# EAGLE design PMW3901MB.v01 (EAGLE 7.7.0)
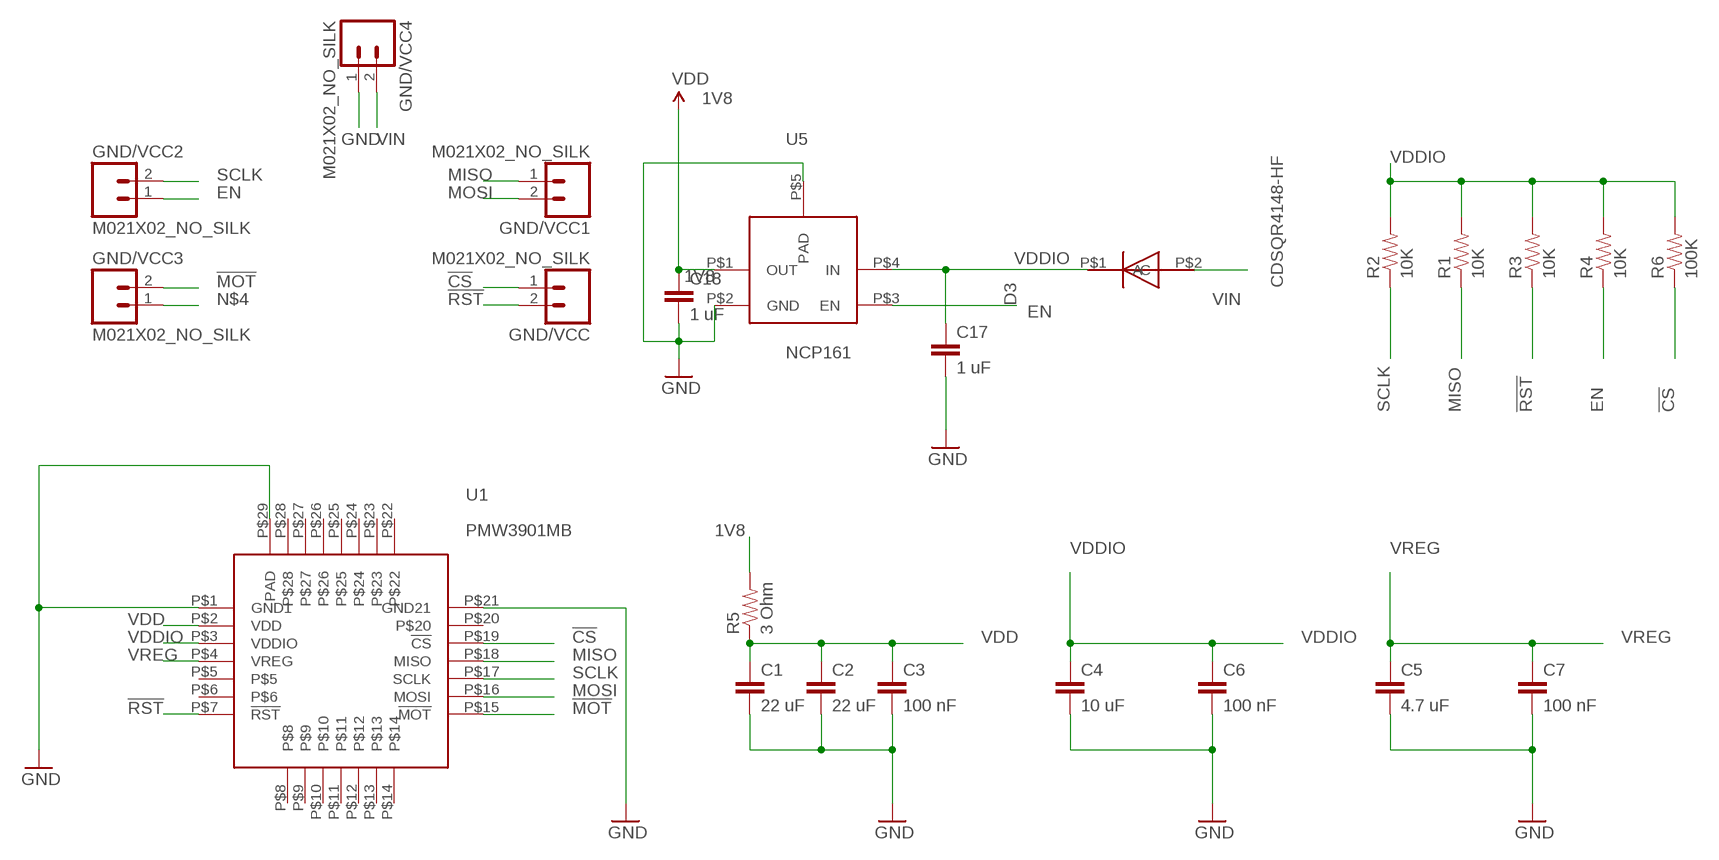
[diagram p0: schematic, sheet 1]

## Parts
C1  22 uF  0402CAP.KW  [0402-CAP@1]
C2  22 uF  0402CAP.KW  [0402-CAP@1]
C3  100 nF  0402CAP.KW  [0402-CAP@1]
C4  10 uF  0402CAP.KW  [0402-CAP@1]
C5  4.7 uF  0402CAP.KW  [0402-CAP@1]
C6  100 nF  0402CAP.KW  [0402-CAP@1]
C7  100 nF  0402CAP.KW  [0402-CAP@1]
C17  1 uF  0402CAP.KW  [0402-CAP@1]
C18  1 uF  0402CAP.KW  [0402-CAP@1]
D3  CDSQR4148-HF  [CDSQR4148-HF]
GND/VCC  M021X02_NO_SILK  [1X02_NO_SILK]
GND/VCC1  M021X02_NO_SILK  [1X02_NO_SILK]
GND/VCC2  M021X02_NO_SILK  [1X02_NO_SILK]
GND/VCC3  M021X02_NO_SILK  [1X02_NO_SILK]
GND/VCC4  M021X02_NO_SILK  [1X02_NO_SILK]
R1  10K  0402RES.KW  [0402-RES]
R2  10K  0402RES.KW  [0402-RES]
R3  10K  0402RES.KW  [0402-RES]
R4  10K  0402RES.KW  [0402-RES]
R5  3 Ohm  0402RES.KW  [0402-RES]
R6  100K  0402RES.KW  [0402-RES]
U1  PMW3901MB  [PMW3901MB]
U5  NCP161  [NCP161]

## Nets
1V8: C18.1 R5.2 U5.P$1(OUT) ; supply symbol labelled VDD
!CS: GND/VCC.1 R6.1 U1.P$19(!CS)
!MOT: GND/VCC3.2 U1.P$15(!MOT)
!RST: GND/VCC.2 R3.1 U1.P$7(!RST)
EN: GND/VCC2.1 R4.1 U5.P$3(EN)
GND: C1.2 C2.2 C3.2 C4.2 C5.2 C6.2 C7.2 C17.2 C18.2 GND/VCC4.1 U1.P$1(GND1) U1.P$21(GND21) U1.P$29(PAD) U5.P$2(GND) U5.P$5(PAD)
MISO: GND/VCC1.1 R1.1 U1.P$18(MISO)
MOSI: GND/VCC1.2 U1.P$16(MOSI)
N$4: GND/VCC3.1
SCLK: GND/VCC2.2 R2.1 U1.P$17(SCLK)
VDD: C1.1 C2.1 C3.1 R5.1 U1.P$2(VDD)
VDDIO: C4.1 C6.1 C17.1 D3.P$1(C) R1.2 R2.2 R3.2 R4.2 R6.2 U1.P$3(VDDIO) U5.P$4(IN)
VIN: D3.P$2(A) GND/VCC4.2
VREG: C5.1 C7.1 U1.P$4(VREG)
Unconnected: U1.P$5 U1.P$6 U1.P$8 U1.P$9 U1.P$10 U1.P$11 U1.P$12 U1.P$13 U1.P$14 U1.P$20 U1.P$22 U1.P$23 U1.P$24 U1.P$25 U1.P$26 U1.P$27 U1.P$28

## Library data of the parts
C1-C7 C17 C18 = SparkFun-Capacitors:0402CAP.KW
D3 = kris:CDSQR4148-HF: ComChip's CDSQR4148-HF high speed 150 mA Io diode
GND/VCC GND/VCC1-GND/VCC4 = SparkFun-Connectors:M02: Standard 2-pin 0.1" header. Use with
R1-R6 = SparkFun-Resistors:0402RES.KW
U1 = kris:PMW3901MB: PMW3901MB flow control camera https://wiki.bitcraze.io/_media/projects:crazyflie2:expansionboards:pot0189-pmw3901mb-txqt-ds-r1.00-200317_20170331160807_public.pdf
U5 = kris:NCP161: NCP161 3V3 LDO voltage regulator

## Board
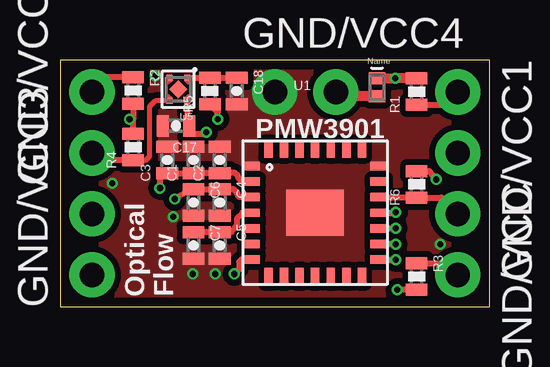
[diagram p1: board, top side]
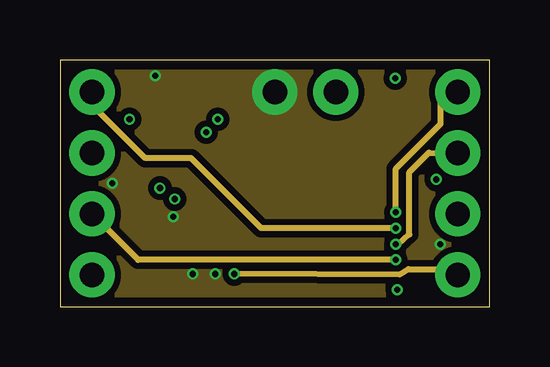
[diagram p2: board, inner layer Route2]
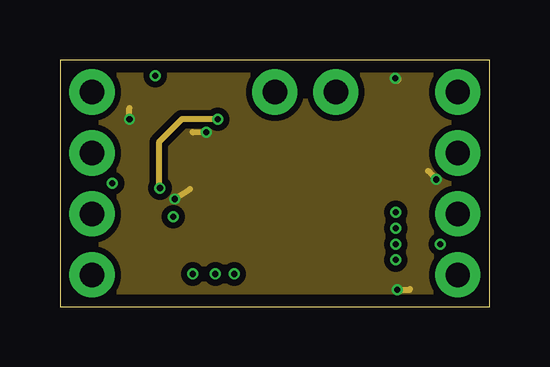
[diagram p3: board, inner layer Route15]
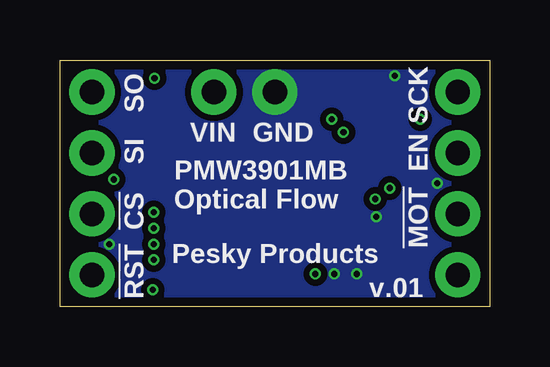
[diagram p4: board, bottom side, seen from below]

Size 17.91 x 10.29 mm. Coordinates in mm from the lower left corner, seen from the top.
Outline: 0,0 17.91,0 17.91,10.29 0,10.29 0,0
Copper layers (1*2*15*16): Top 0.035559375mm / dielectric 0.17018125mm / Route2 0.01778125mm / dielectric 47mil / Route15 0.01778125mm / dielectric 0.17018125mm / Bottom 0.035559375mm
Design rules "OSHPark-4layer *": minimum track width 5mil, minimum drill 10mil, track to track 5mil, track to pad 5mil, pad to pad 5mil, via to via 5mil, smd to smd 5mil, copper to edge 15mil, drill to drill 6mil, minimum pad ring 4mil, minimum via ring 4mil, stop-mask expansion 2.5mil, vias tented up to drill 20mil, thermal gap 10mil

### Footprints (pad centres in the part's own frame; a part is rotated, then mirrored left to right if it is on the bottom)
0402-CAP@1 = smd 0.5 x 0.9: 1 -0.55,0; 2 0.55,0
CDSQR4148-HF = smd 0.7 x 0.5: P$1 0,0.375; P$2 0,-0.375
1X02_NO_SILK = drill 1.016 pad 1.88: 1 0,0; 2 2.54,0
0402-RES = smd 0.5 x 0.9: 1 -0.55,0; 2 0.55,0
PMW3901MB = smd 0.7 x 0.35: P$1 -2.65,1.95; P$2 -2.65,1.3; P$3 -2.65,0.65; P$4 -2.65,0; P$5 -2.65,-0.65; P$6 -2.65,-1.3; P$7 -2.65,-1.95; P$15 2.65,-1.95; P$16 2.65,-1.3; P$17 2.65,-0.65; P$18 2.65,0; P$19 2.65,0.65; P$20 2.65,1.3; P$21 2.65,1.95 | smd 0.35 x 0.7: P$8 -1.95,-2.65; P$9 -1.3,-2.65; P$10 -0.65,-2.65; P$11 0,-2.65; P$12 0.65,-2.65; P$13 1.3,-2.65; P$14 1.95,-2.65; P$22 1.95,2.65; P$23 1.3,2.65; P$24 0.65,2.65; P$25 0,2.65; P$26 -0.65,2.65; P$27 -1.3,2.65; P$28 -1.95,2.65 | smd 2.4 x 1.9: P$29 0,0
NCP161 = smd 0.24 x 0.24: P$1 -0.37,-0.48; P$2 0.37,-0.48; P$3 0.37,0.48; P$4 -0.37,0.48 | smd 0.52 x 0.52 rotated 45: P$5 0,0

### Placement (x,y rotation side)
C1  5.56,6.12 90 top
C2  6.65,6.12 90 top
C3  4.47,6.12 90 top
C4  6.65,4.34 270 top
C5  6.65,2.57 270 top
C6  5.56,4.34 270 top
C7  5.56,2.57 270 top
C17  4.83,7.54 180 top
C18  7.37,8.99 270 top
D3  13.21,9.14 0 top
GND/VCC  16.57,3.87 270 top
GND/VCC1  16.57,8.95 270 top
GND/VCC2  1.33,6.41 90 top
GND/VCC3  1.33,1.33 90 top
GND/VCC4  8.95,8.95 0 top
R1  14.86,8.97 90 top
R2  3.05,9.02 270 top
R3  14.86,1.27 270 top
R4  3.05,6.65 90 top
R5  6.25,8.99 90 top
R6  14.86,5.11 90 top
U1  10.63,3.92 0 top
U5  4.93,9.07 180 top

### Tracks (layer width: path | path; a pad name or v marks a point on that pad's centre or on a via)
1V8
  Top 0.254: U5.P$1 R5.2 C18.1
!CS
  Top 0.254: U1.P$19 14.84,4.57 R6.1 15.89,4.55 GND/VCC.1
!MOT  (via drill 0.25)
  Top 0.254: U1.P$15 13.98,1.97 v13.99,1.96
  Route2 0.254: v13.99,1.96 3.25,1.96 GND/VCC3.2
!RST  (via drill 0.25)
  Top 0.254: R3.1 16.09,1.82 GND/VCC.2 | U1.P$7 7.56,1.97 7.47,1.88 7.47,1.57 v7.26,1.37
  Route2 0.254: v7.26,1.37 14.15,1.35 14.53,1.57 16.33,1.57 GND/VCC.2
EN
  Top 0.203: U5.P$3 3.96,8.59 3.73,8.36 3.73,6.27 3.56,6.11 R4.1
  Top 0.254: R4.1 1.64,6.11 GND/VCC2.1
  Route2 0.254: 1.35,6.43 GND/VCC2.1
GND  (via drill 0.25)
  other vias: 3.96,9.63 15.85,2.62 5.54,1.37 6.48,1.37 4.72,3.76 2.18,5.16
  pour Bottom (isolate 0.254, no thermals): 0,10.29 17.78,10.16 17.78,0 0,0
  pour Top (isolate 0.254, no thermals): 0,10.29 17.78,10.16 17.78,0 0,0
  pour Route2 (isolate 0.254, no thermals): 0,10.29 17.78,10.16 17.78,0 0,0
MISO  (via drill 0.25)
  Top 0.254: R1.1 16.04,8.42 GND/VCC1.1 | U1.P$18 14.11,3.92 v13.99,3.94
  Route2 0.254: v13.99,3.94 13.99,5.77 15.85,7.62 15.85,8.94 16.2,8.59 GND/VCC1.1
MOSI  (via drill 0.25)
  Top 0.254: U1.P$16 13.78,2.62 v13.99,2.62
  Route2 0.254: v13.99,2.62 14.1,2.62 14.55,3.02 14.55,5.61 15.37,6.43 GND/VCC1.2
SCLK  (via drill 0.25)
  Top 0.254: R2.1 1.95,9.57 GND/VCC2.2 | U1.P$17 13.94,3.27 v13.99,3.28
  Route2 0.254: v13.99,3.28 8.38,3.28 5.46,6.2 3.56,6.2 1.4,8.33 1.4,8.89 GND/VCC2.2
VDD  (via drill 0.25)
  Top 0.254: U1.P$2 7.58,5.22 7.42,5.38 7.42,5.46 7.29,5.59 6.7,5.59 C2.1 C1.1 C3.1 4.17,5.41 v4.17,4.95 | v6.58,7.82 6.58,8.11 R5.1
  Route15 0.254: v6.58,7.82 5.08,7.82 4.12,6.86 4.12,5 v4.17,4.95
VDDIO  (via drill 0.25)
  Top 0.203: 5.3,7.65 C17.1
  Top 0.254: U1.P$3 7.49,4.57 7.39,4.67 7.39,4.75 7.24,4.9 6.69,4.9 C4.1 C6.1 5.48,4.89 v4.78,4.5 | R2.2 3.05,7.82 | R3.2 14.03,0.72 v14.05,0.71 | 5.3,7.65 5.3,7.5 5.59,7.21 5.97,7.21 v6.1,7.28 | U5.P$4 5.3,7.62 C17.1 | R4.2 3.05,7.82 | 3.05,7.82 v2.9,7.82 | R6.2 15.38,5.66 v15.67,5.31
  Top 0.406: D3.P$1 v13.96,9.52 v13.97,9.53 13.98,9.52 R1.2
  Route15 0.254: v4.78,4.5 5.41,4.9 | v2.9,7.82 2.9,8.28 | v14.05,0.71 14.55,0.71 14.58,0.74 | v6.1,7.28 5.54,7.26 5.51,7.29 | v15.67,5.31 15.52,5.49 15.34,5.66
  Route15 0.406: v13.97,9.53 13.99,9.53 14.02,9.5
  pour Route15 (isolate 0.254, no thermals): 0.64,9.65 17.27,9.65 17.27,0.64 0.64,0.64
VIN
  Top 0.406: D3.P$2 11.68,8.77 GND/VCC4.2
VREG
  Top 0.254: U1.P$4 7.61,3.92 7.37,3.68 7.37,3.38 7.14,3.12 6.69,3.12 C5.1 C7.1

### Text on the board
tPlace: PMW3901 | Optical / Flow
bPlace: SCK | SO | EN | GND | VIN | SI | !MOT | !CS | PMW3901MB / Optical Flow | !RST | Pesky Products | v.01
